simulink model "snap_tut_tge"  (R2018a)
settings: Solver=VariableStepDiscrete  StartTime=0.0  StopTime=50000  RelTol=1e-3
undefined symbols (not defined in the file): bad_frame, Bit, Both, bram, c, cnt_rst, core_rst, d, data, data_in, eof, eof_in, Falling, hex2dec, ip, ip_in, led, led_rx, led_tx, led_up, link_up, Location, Lower, Minimum_Area, notused, out, overrun, reg, Rising, ROACH2, sfp, SNAP, tx_full, tx_over, Unsigned, Upper, valid, valid_in, Width, xc7k160t
libraries: xbsIndex_r4 x1201, casper_library_misc x9, xps_library x5
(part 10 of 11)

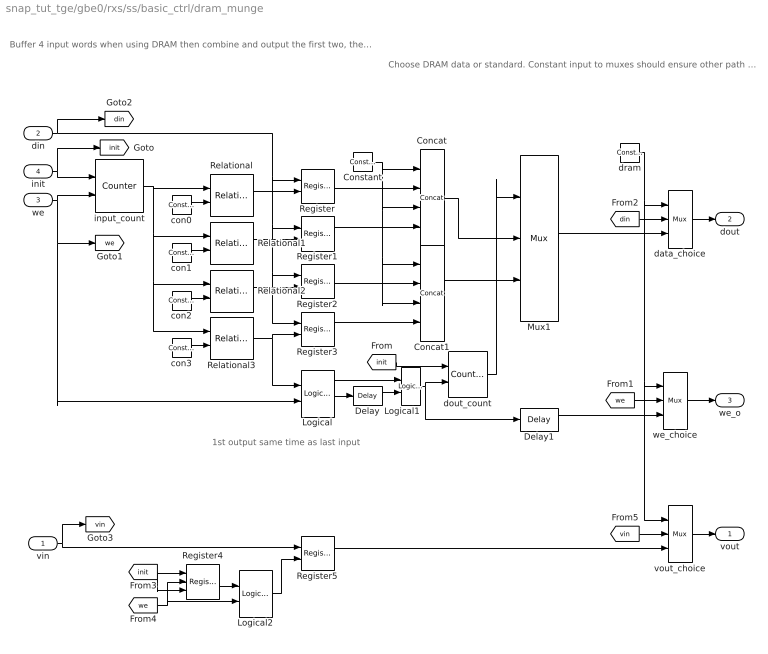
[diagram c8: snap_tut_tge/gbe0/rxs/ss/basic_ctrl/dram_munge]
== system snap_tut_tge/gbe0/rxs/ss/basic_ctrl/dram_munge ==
  note: 1st output same time as last input
  note: Choose DRAM data or standard. Constant input to muxes should ensure other path optimised away
  note: Buffer 4 input words when using DRAM then combine and output the first two, then second. Ensures that a full burst goes through every time so that status register records number of bytes fully in DRAM
  vin : Inport
  din : Inport  Port=2
  we : Inport  Port=3
  init : Inport  Port=4
  Concat : xbsIndex_r4/Concat  num_inputs=4  dbl_ovrd=off  block_type=concat
  Concat1 : xbsIndex_r4/Concat  num_inputs=4  dbl_ovrd=off  block_type=concat
  Constant : xbsIndex_r4/Constant  const=0  gui_display_data_type=Fixed-point  arith_type=Unsigned  n_bits=8  bin_pt=0  preci_type=Single  exp_width=8  frac_width=24  explicit_period=on  period=1  equ=P=C  opselect=C  inp2=PCIN>>17  opr=+  inp1=P  carry=CIN  dbl_ovrd=off  block_type=constant
  Delay : xbsIndex_r4/Delay  rst=off  infoeditControl=Selection of Reset will increase slice count due to use of real FFs and instead of SRLs  en=off  latency=1  reg_retiming=off  dbl_ovrd=off  block_type=delay
  Delay1 : xbsIndex_r4/Delay  rst=off  infoeditControl=Selection of Reset will increase slice count due to use of real FFs and instead of SRLs  en=off  latency=1  reg_retiming=off  dbl_ovrd=off  block_type=delay
  Logical : xbsIndex_r4/Logical  logical_function=AND  inputs=2  en=off  latency=1  precision=Full  arith_type=Unsigned  n_bits=16  bin_pt=0  align_bp=on  dbl_ovrd=off  block_type=logical
  Logical1 : xbsIndex_r4/Logical  logical_function=OR  inputs=2  en=off  latency=0  precision=Full  arith_type=Unsigned  n_bits=16  bin_pt=0  align_bp=on  dbl_ovrd=off  block_type=logical
  Logical2 : xbsIndex_r4/Logical  logical_function=AND  inputs=2  en=off  latency=0  precision=Full  arith_type=Unsigned  n_bits=16  bin_pt=0  align_bp=on  dbl_ovrd=off  block_type=logical
  Mux1 : xbsIndex_r4/Mux  inputs=2  en=off  latency=1  precision=Full  arith_type=Unsigned  n_bits=16  bin_pt=14  quantization=Truncate  overflow=Wrap  dbl_ovrd=off  block_type=mux
  Register{,1..3,5} (5 alike) : xbsIndex_r4/Register  init=0  rst=off  en=on  dbl_ovrd=off  block_type=register
  Register4 : xbsIndex_r4/Register  init=0  rst=on  en=on  dbl_ovrd=off  block_type=register
  Relational{,1..3} (4 alike) : xbsIndex_r4/Relational  mode=a=b  op_type=Bool  en=off  latency=0  dbl_ovrd=off  block_type=relational
  con0 : xbsIndex_r4/Constant  const=0  gui_display_data_type=Fixed-point  arith_type=Unsigned  n_bits=2  bin_pt=0  preci_type=Single  exp_width=8  frac_width=24  explicit_period=on  period=1  equ=P=C  opselect=C  inp2=PCIN>>17  opr=+  inp1=P  carry=CIN  dbl_ovrd=off  block_type=constant
  con1 : xbsIndex_r4/Constant  const=1  gui_display_data_type=Fixed-point  arith_type=Unsigned  n_bits=2  bin_pt=0  preci_type=Single  exp_width=8  frac_width=24  explicit_period=on  period=1  equ=P=C  opselect=C  inp2=PCIN>>17  opr=+  inp1=P  carry=CIN  dbl_ovrd=off  block_type=constant
  con2 : xbsIndex_r4/Constant  const=2  gui_display_data_type=Fixed-point  arith_type=Unsigned  n_bits=2  bin_pt=0  preci_type=Single  exp_width=8  frac_width=24  explicit_period=on  period=1  equ=P=C  opselect=C  inp2=PCIN>>17  opr=+  inp1=P  carry=CIN  dbl_ovrd=off  block_type=constant
  con3 : xbsIndex_r4/Constant  const=3  gui_display_data_type=Fixed-point  arith_type=Unsigned  n_bits=2  bin_pt=0  preci_type=Single  exp_width=8  frac_width=24  explicit_period=on  period=1  equ=P=C  opselect=C  inp2=PCIN>>17  opr=+  inp1=P  carry=CIN  dbl_ovrd=off  block_type=constant
  data_choice : xbsIndex_r4/Mux  inputs=2  en=off  latency=0  precision=User Defined  arith_type=Unsigned  n_bits=128  bin_pt=0  quantization=Truncate  overflow=Wrap  dbl_ovrd=off  block_type=mux
  dout_count : xbsIndex_r4/Counter  cnt_type=Free Running  cnt_to=Inf  operation=Up  start_count=0  cnt_by_val=1  arith_type=Unsigned  n_bits=1  bin_pt=0  load_pin=off  rst=on  en=on  explicit_period=on  period=1  use_behavioral_HDL=off  implementation=Fabric  dbl_ovrd=off  block_type=counter
  dram : xbsIndex_r4/Constant  const=0  gui_display_data_type=Fixed-point  arith_type=Boolean  n_bits=16  bin_pt=14  preci_type=Single  exp_width=8  frac_width=24  explicit_period=on  period=1  equ=P=C  opselect=C  inp2=PCIN>>17  opr=+  inp1=P  carry=CIN  dbl_ovrd=off  block_type=constant
  input_count : xbsIndex_r4/Counter  cnt_type=Free Running  cnt_to=Inf  operation=Up  start_count=0  cnt_by_val=1  arith_type=Unsigned  n_bits=2  bin_pt=0  load_pin=off  rst=on  en=on  explicit_period=on  period=1  use_behavioral_HDL=off  implementation=Fabric  dbl_ovrd=off  block_type=counter
  vout_choice : xbsIndex_r4/Mux  inputs=2  en=off  latency=0  precision=Full  arith_type=Unsigned  n_bits=16  bin_pt=14  quantization=Truncate  overflow=Wrap  dbl_ovrd=off  block_type=mux
  we_choice : xbsIndex_r4/Mux  inputs=2  en=off  latency=0  precision=Full  arith_type=Unsigned  n_bits=16  bin_pt=14  quantization=Truncate  overflow=Wrap  dbl_ovrd=off  block_type=mux
  vout : Outport
  dout : Outport  Port=2
  we_o : Outport  Port=3
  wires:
  Register3/1 -> Concat1/4
  Register2/1 -> Concat1/2
  Constant/1 -> Concat1/3, Concat1/1, Concat/3, Concat/1
  Register1/1 -> Concat/4
  Register/1 -> Concat/2
  [vin] -> vout_choice/2
  Register5/1 -> vout_choice/3
  vout_choice/1 -> vout/1
  Logical2/1 -> Register5/2
  [we] -> Logical2/2, Register4/2
  vin/1 -> [vin], Register5/1
  Register4/1 -> Logical2/1
  [init] -> Register4/3, Register4/1
  dram/1 -> vout_choice/1, we_choice/1, data_choice/1
  [din] -> data_choice/2
  Mux1/1 -> data_choice/3
  [we] -> we_choice/2
  Delay1/1 -> we_choice/3
  we_choice/1 -> we_o/1
  dout_count/1 -> Mux1/1
  [init] -> dout_count/1
  Logical1/1 -> Delay1/1, dout_count/2
  Concat1/1 -> Mux1/3
  Concat/1 -> Mux1/2
  Delay/1 -> Logical1/2
  Logical/1 -> Logical1/1, Delay/1
  Relational3/1 -> Logical/1, Register3/2
  Relational2/1 -> Register2/2
  Relational1/1 -> Register1/2
  Relational/1 -> Register/2
  con3/1 -> Relational3/2
  con2/1 -> Relational2/2
  con1/1 -> Relational1/2
  con0/1 -> Relational/2
  input_count/1 -> Relational3/1, Relational2/1, Relational1/1, Relational/1
  din/1 -> [din], Register3/1, Register2/1, Register1/1, Register/1
  we/1 -> [we], Logical/2, input_count/2
  init/1 -> [init], input_count/1
  data_choice/1 -> dout/1

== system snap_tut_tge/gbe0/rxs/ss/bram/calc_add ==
  note: If reading/writing words smaller than 32 bits, change address so that addressing is big endian instead of little, otherwise pass through
  note: Use behavioural HDL so that gets optimised to minimum logic
  in : Inport
  add_sub : xbsIndex_r4/AddSub  mode=Subtraction  use_carryin=off  use_carryout=off  en=off  latency=0  precision=User Defined  arith_type=Unsigned  n_bits=max(1, log2(32/data_width))  bin_pt=0  quantization=Truncate  overflow=Wrap  use_behavioral_HDL=on  hw_selection=Fabric  pipelined=off  dbl_ovrd=off  block_type=addsub
  concat : xbsIndex_r4/Concat  num_inputs=2  dbl_ovrd=off  block_type=concat
  const : xbsIndex_r4/Constant  const=max(0, 32/data_width-1)  gui_display_data_type=Fixed-point  arith_type=Unsigned  n_bits=max(1, log2(32/data_width))  bin_pt=0  preci_type=Single  exp_width=8  frac_width=24  explicit_period=on  period=sample_rate  equ=P=C  opselect=C  inp2=PCIN>>17  opr=+  inp1=P  carry=CIN  dbl_ovrd=off  block_type=constant
  convert_addr : xbsIndex_r4/Convert  gui_display_data_type=Fixed-point  arith_type=Unsigned  n_bits=addr_width  bin_pt=0  float_type=Single  exp_bits=8  fraction_bits=24  quantization=Truncate  overflow=Wrap  en=off  latency=0  pipeline=off  dbl_ovrd=off  block_type=convert
  lsw : xbsIndex_r4/Slice  nbits=max(1, log2(32/data_width))  boolean_output=off  mode=Lower Bit Location + Width  bit1=0  base1=MSB of Input  bit0=0  base0=LSB of Input  dbl_ovrd=off  block_type=slice
  manipulate : xbsIndex_r4/Constant  const=min(1, floor(32/data_width) - 1)  gui_display_data_type=Fixed-point  arith_type=Unsigned  n_bits=1  bin_pt=0  preci_type=Single  exp_width=8  frac_width=24  explicit_period=on  period=sample_rate  equ=P=C  opselect=C  inp2=PCIN>>17  opr=+  inp1=P  carry=CIN  dbl_ovrd=off  block_type=constant
  msw : xbsIndex_r4/Slice  nbits=addr_width - max(1, log2(32/data_width))  boolean_output=off  mode=Upper Bit Location + Width  bit1=0  base1=MSB of Input  bit0=0  base0=LSB of Input  dbl_ovrd=off  block_type=slice
  mux : xbsIndex_r4/Mux  inputs=2  en=off  latency=0  precision=Full  arith_type=Unsigned  n_bits=16  bin_pt=14  quantization=Truncate  overflow=Wrap  dbl_ovrd=off  block_type=mux
  out : Outport
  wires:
  in/1 -> convert_addr/1
  add_sub/1 -> concat/2
  msw/1 -> concat/1
  concat/1 -> mux/3
  manipulate/1 -> mux/1
  mux/1 -> out/1
  lsw/1 -> add_sub/2
  const/1 -> add_sub/1
  convert_addr/1 -> lsw/1, msw/1, mux/2

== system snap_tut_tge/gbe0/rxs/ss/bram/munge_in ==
  din : Inport
  join : Subsystem  AncestorBlock=casper_library_flow_control/bus_create  mask(bus_create){inputNum=4}
      mask prompts: inputNum "Number of inputs:"
      mask init:
      | bus_create_init(gcb,...
      |     'inputNum', inputNum);
  reinterpret : xbsIndex_r4/Reinterpret  force_arith_type=on  arith_type=Unsigned  force_bin_pt=on  bin_pt=0  block_type=reinterpret
  reinterpret_out : xbsIndex_r4/Reinterpret  force_arith_type=on  arith_type=Unsigned  force_bin_pt=on  bin_pt=0  block_type=reinterpret
  split : Subsystem  AncestorBlock=casper_library_flow_control/bus_expand  mask(bus_expand){mode=divisions of arbitrary size, outputNum=1, outputWidth=[32 32 32 32], outputBinaryPt=[0 0 0 0], outputArithmeticType=[0 0 0 0], show_format=off, outputToWorkspace=off, variablePrefix=out, outputToModelAsWell=on}
      mask prompts: outputNum "Number of outputs:"; outputWidth "Output width [msb ... lsb]:"; outputBinaryPt "Output binary point position [msb ... lsb]:"; outputArithmeticType "Output arithmetic type (ufix=0, fix=1, bool=2) [msb ... lsb]:"; show_format "Print format string?"; outputToWorkspace "Output to workspace?"; variablePrefix "Variable name prefix:"; outputToModelAsWell "Output to model as well?"
      mask help: Expands a 'bus' made using a bus_create or Xilinx concat block. The input will be divided into the specified number of outputs with the specified arithmetic types. Divisions are made from most significant bit.
      mask init:
      | bus_expand_init(gcb,...
      |     'mode', mode, ...
      |     'outputNum', outputNum, ...
      |     'outputWidth', outputWidth, ...
      |     'outputBinaryPt', outputBinaryPt, ...
      |     'outputArithmeticType', outputArithmeticType, ...
      |     'show_format', show_format, ...
      |     'outputToWorkspace', outputToWorkspace, ...
      |     'variablePrefix', variablePrefix, ...
      |     'outputToModelAsWell', outputToModelAsWell);
  dout : Outport
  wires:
  reinterpret_out/1 -> dout/1
  din/1 -> reinterpret/1
  reinterpret/1 -> split/1(bus_in)
  join/1(bus_out) -> reinterpret_out/1
  split/4(lsb_out1) -> join/1(in1)
  split/3(out2) -> join/2(in2)
  split/2(out3) -> join/3(in3)
  split/1(msb_out4) -> join/4(in4)

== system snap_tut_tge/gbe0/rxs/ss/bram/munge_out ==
  din : Inport
  join : Subsystem  AncestorBlock=casper_library_flow_control/bus_create  mask(bus_create){inputNum=4}
      mask prompts: inputNum "Number of inputs:"
      mask init:
      | bus_create_init(gcb,...
      |     'inputNum', inputNum);
  reinterpret : xbsIndex_r4/Reinterpret  force_arith_type=on  arith_type=Unsigned  force_bin_pt=on  bin_pt=0  block_type=reinterpret
  reinterpret_out : xbsIndex_r4/Reinterpret  force_arith_type=on  arith_type=Unsigned  force_bin_pt=on  bin_pt=0  block_type=reinterpret
  split : Subsystem  AncestorBlock=casper_library_flow_control/bus_expand  mask(bus_expand){mode=divisions of arbitrary size, outputNum=1, outputWidth=[32 32 32 32], outputBinaryPt=[0 0 0 0], outputArithmeticType=[0 0 0 0], show_format=off, outputToWorkspace=off, variablePrefix=out, outputToModelAsWell=on}
      mask prompts: outputNum "Number of outputs:"; outputWidth "Output width [msb ... lsb]:"; outputBinaryPt "Output binary point position [msb ... lsb]:"; outputArithmeticType "Output arithmetic type (ufix=0, fix=1, bool=2) [msb ... lsb]:"; show_format "Print format string?"; outputToWorkspace "Output to workspace?"; variablePrefix "Variable name prefix:"; outputToModelAsWell "Output to model as well?"
      mask help: Expands a 'bus' made using a bus_create or Xilinx concat block. The input will be divided into the specified number of outputs with the specified arithmetic types. Divisions are made from most significant bit.
      mask init:
      | bus_expand_init(gcb,...
      |     'mode', mode, ...
      |     'outputNum', outputNum, ...
      |     'outputWidth', outputWidth, ...
      |     'outputBinaryPt', outputBinaryPt, ...
      |     'outputArithmeticType', outputArithmeticType, ...
      |     'show_format', show_format, ...
      |     'outputToWorkspace', outputToWorkspace, ...
      |     'variablePrefix', variablePrefix, ...
      |     'outputToModelAsWell', outputToModelAsWell);
  dout : Outport
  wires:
  reinterpret_out/1 -> dout/1
  din/1 -> reinterpret/1
  reinterpret/1 -> split/1(bus_in)
  join/1(bus_out) -> reinterpret_out/1
  split/4(lsb_out1) -> join/1(in1)
  split/3(out2) -> join/2(in2)
  split/2(out3) -> join/3(in3)
  split/1(msb_out4) -> join/4(in4)

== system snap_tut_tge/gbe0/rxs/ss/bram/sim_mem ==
  addr : Inport
  data : Inport  Port=2
  we : Inport  Port=3
  Data Type Conversion : DataTypeConversion  OutDataTypeStr=single
  Data Type Conversion1 : DataTypeConversion  OutDataTypeStr=double
  Data Type Conversion2 : DataTypeConversion  OutDataTypeStr=boolean
  sfunc : M-S-Function  FunctionName=shared_bram_sim_sfunc  Parameters=depth_bits, latency, init_vals  mask{depth_bits=addr_width, latency=csp_latency, init_vals=init_vals}
      mask prompts: depth_bits "Depth (2^?):"; latency "Latency (>=1):"; init_vals "Initial values:"
  sim_addr : xbsIndex_r4/Gateway Out  inherit_from_input=off  hdl_port=off  rows=1  columns=1  UseAsDAC=off  DACChannel='1'  interface=None  automatic_assignment=on  address_offset=hex2dec('00')  intf_name=''  intf_description=''  timing_constraint=None  locs_specified=off  LOCs={}  io_standard={}  block_type=gatewayout
  sim_data : xbsIndex_r4/Gateway Out  inherit_from_input=off  hdl_port=off  rows=1  columns=1  UseAsDAC=off  DACChannel='1'  interface=None  automatic_assignment=on  address_offset=hex2dec('00')  intf_name=''  intf_description=''  timing_constraint=None  locs_specified=off  LOCs={}  io_standard={}  block_type=gatewayout
  sim_we : xbsIndex_r4/Gateway Out  inherit_from_input=off  hdl_port=off  rows=1  columns=1  UseAsDAC=off  DACChannel='1'  interface=None  automatic_assignment=on  address_offset=hex2dec('00')  intf_name=''  intf_description=''  timing_constraint=None  locs_specified=off  LOCs={}  io_standard={}  block_type=gatewayout
  data_out : Outport
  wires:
  addr/1 -> sim_addr/1
  data/1 -> sim_data/1
  we/1 -> sim_we/1
  sim_addr/1 -> Data Type Conversion/1
  sim_data/1 -> Data Type Conversion1/1
  sim_we/1 -> Data Type Conversion2/1
  Data Type Conversion/1 -> sfunc/1  "addr"
  Data Type Conversion1/1 -> sfunc/2  "data_in"
  Data Type Conversion2/1 -> sfunc/3  "we"
  sfunc/1 -> data_out/1  "output"

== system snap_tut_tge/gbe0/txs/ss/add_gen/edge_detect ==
  in : Inport
  Delay : xbsIndex_r4/Delay  rst=off  infoeditControl=Selection of Reset will increase slice count due to use of real FFs and instead of SRLs  en=off  latency=1  reg_retiming=off  dbl_ovrd=off  block_type=delay
  Inverter : xbsIndex_r4/Inverter  en=off  latency=0  dbl_ovrd=off  block_type=inv
  edge_op : xbsIndex_r4/Logical  logical_function=XNOR  inputs=2  en=off  latency=0  precision=Full  arith_type=Unsigned  n_bits=8  bin_pt=2  align_bp=on  dbl_ovrd=off  block_type=logical
  out : Outport
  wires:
  Delay/1 -> edge_op/2
  in/1 -> Delay/1, Inverter/1
  edge_op/1 -> out/1
  Inverter/1 -> edge_op/1

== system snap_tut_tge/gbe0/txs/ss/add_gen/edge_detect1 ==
  in : Inport
  Delay : xbsIndex_r4/Delay  rst=off  infoeditControl=Selection of Reset will increase slice count due to use of real FFs and instead of SRLs  en=off  latency=1  reg_retiming=off  dbl_ovrd=off  block_type=delay
  Inverter : xbsIndex_r4/Inverter  en=off  latency=0  dbl_ovrd=off  block_type=inv
  edge_op : xbsIndex_r4/Logical  logical_function=XNOR  inputs=2  en=off  latency=0  precision=Full  arith_type=Unsigned  n_bits=8  bin_pt=2  align_bp=on  dbl_ovrd=off  block_type=logical
  out : Outport
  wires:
  Inverter/1 -> edge_op/1
  edge_op/1 -> out/1
  in/1 -> Inverter/1, Delay/1
  Delay/1 -> edge_op/2

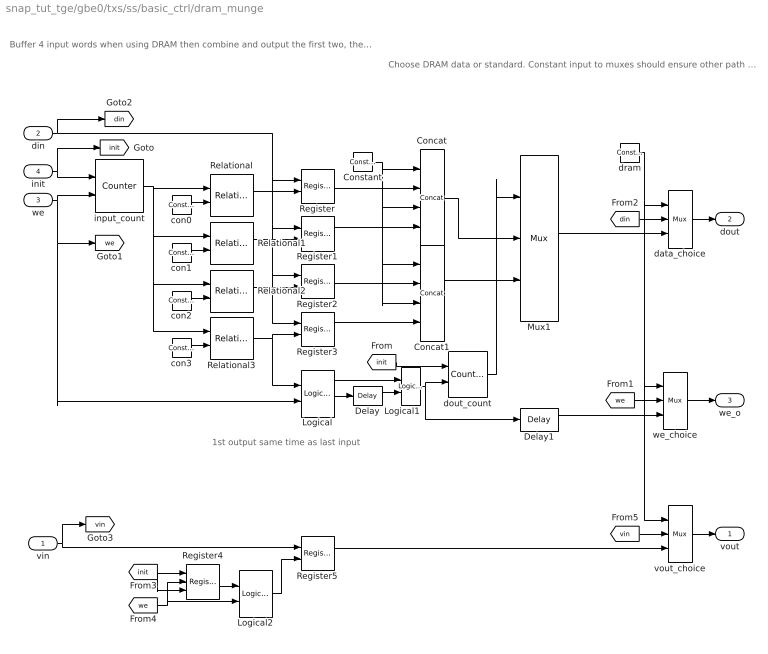
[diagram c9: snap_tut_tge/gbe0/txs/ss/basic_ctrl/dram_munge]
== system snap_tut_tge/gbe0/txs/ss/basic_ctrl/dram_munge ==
  note: 1st output same time as last input
  note: Choose DRAM data or standard. Constant input to muxes should ensure other path optimised away
  note: Buffer 4 input words when using DRAM then combine and output the first two, then second. Ensures that a full burst goes through every time so that status register records number of bytes fully in DRAM
  vin : Inport
  din : Inport  Port=2
  we : Inport  Port=3
  init : Inport  Port=4
  Concat : xbsIndex_r4/Concat  num_inputs=4  dbl_ovrd=off  block_type=concat
  Concat1 : xbsIndex_r4/Concat  num_inputs=4  dbl_ovrd=off  block_type=concat
  Constant : xbsIndex_r4/Constant  const=0  gui_display_data_type=Fixed-point  arith_type=Unsigned  n_bits=8  bin_pt=0  preci_type=Single  exp_width=8  frac_width=24  explicit_period=on  period=1  equ=P=C  opselect=C  inp2=PCIN>>17  opr=+  inp1=P  carry=CIN  dbl_ovrd=off  block_type=constant
  Delay : xbsIndex_r4/Delay  rst=off  infoeditControl=Selection of Reset will increase slice count due to use of real FFs and instead of SRLs  en=off  latency=1  reg_retiming=off  dbl_ovrd=off  block_type=delay
  Delay1 : xbsIndex_r4/Delay  rst=off  infoeditControl=Selection of Reset will increase slice count due to use of real FFs and instead of SRLs  en=off  latency=1  reg_retiming=off  dbl_ovrd=off  block_type=delay
  Logical : xbsIndex_r4/Logical  logical_function=AND  inputs=2  en=off  latency=1  precision=Full  arith_type=Unsigned  n_bits=16  bin_pt=0  align_bp=on  dbl_ovrd=off  block_type=logical
  Logical1 : xbsIndex_r4/Logical  logical_function=OR  inputs=2  en=off  latency=0  precision=Full  arith_type=Unsigned  n_bits=16  bin_pt=0  align_bp=on  dbl_ovrd=off  block_type=logical
  Logical2 : xbsIndex_r4/Logical  logical_function=AND  inputs=2  en=off  latency=0  precision=Full  arith_type=Unsigned  n_bits=16  bin_pt=0  align_bp=on  dbl_ovrd=off  block_type=logical
  Mux1 : xbsIndex_r4/Mux  inputs=2  en=off  latency=1  precision=Full  arith_type=Unsigned  n_bits=16  bin_pt=14  quantization=Truncate  overflow=Wrap  dbl_ovrd=off  block_type=mux
  Register{,1..3,5} (5 alike) : xbsIndex_r4/Register  init=0  rst=off  en=on  dbl_ovrd=off  block_type=register
  Register4 : xbsIndex_r4/Register  init=0  rst=on  en=on  dbl_ovrd=off  block_type=register
  Relational{,1..3} (4 alike) : xbsIndex_r4/Relational  mode=a=b  op_type=Bool  en=off  latency=0  dbl_ovrd=off  block_type=relational
  con0 : xbsIndex_r4/Constant  const=0  gui_display_data_type=Fixed-point  arith_type=Unsigned  n_bits=2  bin_pt=0  preci_type=Single  exp_width=8  frac_width=24  explicit_period=on  period=1  equ=P=C  opselect=C  inp2=PCIN>>17  opr=+  inp1=P  carry=CIN  dbl_ovrd=off  block_type=constant
  con1 : xbsIndex_r4/Constant  const=1  gui_display_data_type=Fixed-point  arith_type=Unsigned  n_bits=2  bin_pt=0  preci_type=Single  exp_width=8  frac_width=24  explicit_period=on  period=1  equ=P=C  opselect=C  inp2=PCIN>>17  opr=+  inp1=P  carry=CIN  dbl_ovrd=off  block_type=constant
  con2 : xbsIndex_r4/Constant  const=2  gui_display_data_type=Fixed-point  arith_type=Unsigned  n_bits=2  bin_pt=0  preci_type=Single  exp_width=8  frac_width=24  explicit_period=on  period=1  equ=P=C  opselect=C  inp2=PCIN>>17  opr=+  inp1=P  carry=CIN  dbl_ovrd=off  block_type=constant
  con3 : xbsIndex_r4/Constant  const=3  gui_display_data_type=Fixed-point  arith_type=Unsigned  n_bits=2  bin_pt=0  preci_type=Single  exp_width=8  frac_width=24  explicit_period=on  period=1  equ=P=C  opselect=C  inp2=PCIN>>17  opr=+  inp1=P  carry=CIN  dbl_ovrd=off  block_type=constant
  data_choice : xbsIndex_r4/Mux  inputs=2  en=off  latency=0  precision=User Defined  arith_type=Unsigned  n_bits=128  bin_pt=0  quantization=Truncate  overflow=Wrap  dbl_ovrd=off  block_type=mux
  dout_count : xbsIndex_r4/Counter  cnt_type=Free Running  cnt_to=Inf  operation=Up  start_count=0  cnt_by_val=1  arith_type=Unsigned  n_bits=1  bin_pt=0  load_pin=off  rst=on  en=on  explicit_period=on  period=1  use_behavioral_HDL=off  implementation=Fabric  dbl_ovrd=off  block_type=counter
  dram : xbsIndex_r4/Constant  const=0  gui_display_data_type=Fixed-point  arith_type=Boolean  n_bits=16  bin_pt=14  preci_type=Single  exp_width=8  frac_width=24  explicit_period=on  period=1  equ=P=C  opselect=C  inp2=PCIN>>17  opr=+  inp1=P  carry=CIN  dbl_ovrd=off  block_type=constant
  input_count : xbsIndex_r4/Counter  cnt_type=Free Running  cnt_to=Inf  operation=Up  start_count=0  cnt_by_val=1  arith_type=Unsigned  n_bits=2  bin_pt=0  load_pin=off  rst=on  en=on  explicit_period=on  period=1  use_behavioral_HDL=off  implementation=Fabric  dbl_ovrd=off  block_type=counter
  vout_choice : xbsIndex_r4/Mux  inputs=2  en=off  latency=0  precision=Full  arith_type=Unsigned  n_bits=16  bin_pt=14  quantization=Truncate  overflow=Wrap  dbl_ovrd=off  block_type=mux
  we_choice : xbsIndex_r4/Mux  inputs=2  en=off  latency=0  precision=Full  arith_type=Unsigned  n_bits=16  bin_pt=14  quantization=Truncate  overflow=Wrap  dbl_ovrd=off  block_type=mux
  vout : Outport
  dout : Outport  Port=2
  we_o : Outport  Port=3
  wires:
  Register3/1 -> Concat1/4
  Register2/1 -> Concat1/2
  Constant/1 -> Concat1/3, Concat1/1, Concat/3, Concat/1
  Register1/1 -> Concat/4
  Register/1 -> Concat/2
  [vin] -> vout_choice/2
  Register5/1 -> vout_choice/3
  vout_choice/1 -> vout/1
  Logical2/1 -> Register5/2
  [we] -> Logical2/2, Register4/2
  vin/1 -> [vin], Register5/1
  Register4/1 -> Logical2/1
  [init] -> Register4/3, Register4/1
  dram/1 -> vout_choice/1, we_choice/1, data_choice/1
  [din] -> data_choice/2
  Mux1/1 -> data_choice/3
  [we] -> we_choice/2
  Delay1/1 -> we_choice/3
  we_choice/1 -> we_o/1
  dout_count/1 -> Mux1/1
  [init] -> dout_count/1
  Logical1/1 -> Delay1/1, dout_count/2
  Concat1/1 -> Mux1/3
  Concat/1 -> Mux1/2
  Delay/1 -> Logical1/2
  Logical/1 -> Logical1/1, Delay/1
  Relational3/1 -> Logical/1, Register3/2
  Relational2/1 -> Register2/2
  Relational1/1 -> Register1/2
  Relational/1 -> Register/2
  con3/1 -> Relational3/2
  con2/1 -> Relational2/2
  con1/1 -> Relational1/2
  con0/1 -> Relational/2
  input_count/1 -> Relational3/1, Relational2/1, Relational1/1, Relational/1
  din/1 -> [din], Register3/1, Register2/1, Register1/1, Register/1
  we/1 -> [we], Logical/2, input_count/2
  init/1 -> [init], input_count/1
  data_choice/1 -> dout/1

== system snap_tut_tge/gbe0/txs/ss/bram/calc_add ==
  note: If reading/writing words smaller than 32 bits, change address so that addressing is big endian instead of little, otherwise pass through
  note: Use behavioural HDL so that gets optimised to minimum logic
  in : Inport
  add_sub : xbsIndex_r4/AddSub  mode=Subtraction  use_carryin=off  use_carryout=off  en=off  latency=0  precision=User Defined  arith_type=Unsigned  n_bits=max(1, log2(32/data_width))  bin_pt=0  quantization=Truncate  overflow=Wrap  use_behavioral_HDL=on  hw_selection=Fabric  pipelined=off  dbl_ovrd=off  block_type=addsub
  concat : xbsIndex_r4/Concat  num_inputs=2  dbl_ovrd=off  block_type=concat
  const : xbsIndex_r4/Constant  const=max(0, 32/data_width-1)  gui_display_data_type=Fixed-point  arith_type=Unsigned  n_bits=max(1, log2(32/data_width))  bin_pt=0  preci_type=Single  exp_width=8  frac_width=24  explicit_period=on  period=sample_rate  equ=P=C  opselect=C  inp2=PCIN>>17  opr=+  inp1=P  carry=CIN  dbl_ovrd=off  block_type=constant
  convert_addr : xbsIndex_r4/Convert  gui_display_data_type=Fixed-point  arith_type=Unsigned  n_bits=addr_width  bin_pt=0  float_type=Single  exp_bits=8  fraction_bits=24  quantization=Truncate  overflow=Wrap  en=off  latency=0  pipeline=off  dbl_ovrd=off  block_type=convert
  lsw : xbsIndex_r4/Slice  nbits=max(1, log2(32/data_width))  boolean_output=off  mode=Lower Bit Location + Width  bit1=0  base1=MSB of Input  bit0=0  base0=LSB of Input  dbl_ovrd=off  block_type=slice
  manipulate : xbsIndex_r4/Constant  const=min(1, floor(32/data_width) - 1)  gui_display_data_type=Fixed-point  arith_type=Unsigned  n_bits=1  bin_pt=0  preci_type=Single  exp_width=8  frac_width=24  explicit_period=on  period=sample_rate  equ=P=C  opselect=C  inp2=PCIN>>17  opr=+  inp1=P  carry=CIN  dbl_ovrd=off  block_type=constant
  msw : xbsIndex_r4/Slice  nbits=addr_width - max(1, log2(32/data_width))  boolean_output=off  mode=Upper Bit Location + Width  bit1=0  base1=MSB of Input  bit0=0  base0=LSB of Input  dbl_ovrd=off  block_type=slice
  mux : xbsIndex_r4/Mux  inputs=2  en=off  latency=0  precision=Full  arith_type=Unsigned  n_bits=16  bin_pt=14  quantization=Truncate  overflow=Wrap  dbl_ovrd=off  block_type=mux
  out : Outport
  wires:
  in/1 -> convert_addr/1
  add_sub/1 -> concat/2
  msw/1 -> concat/1
  concat/1 -> mux/3
  manipulate/1 -> mux/1
  mux/1 -> out/1
  lsw/1 -> add_sub/2
  const/1 -> add_sub/1
  convert_addr/1 -> lsw/1, msw/1, mux/2

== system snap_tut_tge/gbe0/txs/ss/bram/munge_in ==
  din : Inport
  join : Subsystem  AncestorBlock=casper_library_flow_control/bus_create  mask(bus_create){inputNum=4}
      mask prompts: inputNum "Number of inputs:"
      mask init:
      | bus_create_init(gcb,...
      |     'inputNum', inputNum);
  reinterpret : xbsIndex_r4/Reinterpret  force_arith_type=on  arith_type=Unsigned  force_bin_pt=on  bin_pt=0  block_type=reinterpret
  reinterpret_out : xbsIndex_r4/Reinterpret  force_arith_type=on  arith_type=Unsigned  force_bin_pt=on  bin_pt=0  block_type=reinterpret
  split : Subsystem  AncestorBlock=casper_library_flow_control/bus_expand  mask(bus_expand){mode=divisions of arbitrary size, outputNum=1, outputWidth=[32 32 32 32], outputBinaryPt=[0 0 0 0], outputArithmeticType=[0 0 0 0], show_format=off, outputToWorkspace=off, variablePrefix=out, outputToModelAsWell=on}
      mask prompts: outputNum "Number of outputs:"; outputWidth "Output width [msb ... lsb]:"; outputBinaryPt "Output binary point position [msb ... lsb]:"; outputArithmeticType "Output arithmetic type (ufix=0, fix=1, bool=2) [msb ... lsb]:"; show_format "Print format string?"; outputToWorkspace "Output to workspace?"; variablePrefix "Variable name prefix:"; outputToModelAsWell "Output to model as well?"
      mask help: Expands a 'bus' made using a bus_create or Xilinx concat block. The input will be divided into the specified number of outputs with the specified arithmetic types. Divisions are made from most significant bit.
      mask init:
      | bus_expand_init(gcb,...
      |     'mode', mode, ...
      |     'outputNum', outputNum, ...
      |     'outputWidth', outputWidth, ...
      |     'outputBinaryPt', outputBinaryPt, ...
      |     'outputArithmeticType', outputArithmeticType, ...
      |     'show_format', show_format, ...
      |     'outputToWorkspace', outputToWorkspace, ...
      |     'variablePrefix', variablePrefix, ...
      |     'outputToModelAsWell', outputToModelAsWell);
  dout : Outport
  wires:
  reinterpret_out/1 -> dout/1
  din/1 -> reinterpret/1
  reinterpret/1 -> split/1(bus_in)
  join/1(bus_out) -> reinterpret_out/1
  split/4(lsb_out1) -> join/1(in1)
  split/3(out2) -> join/2(in2)
  split/2(out3) -> join/3(in3)
  split/1(msb_out4) -> join/4(in4)

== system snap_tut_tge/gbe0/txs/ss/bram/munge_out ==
  din : Inport
  join : Subsystem  AncestorBlock=casper_library_flow_control/bus_create  mask(bus_create){inputNum=4}
      mask prompts: inputNum "Number of inputs:"
      mask init:
      | bus_create_init(gcb,...
      |     'inputNum', inputNum);
  reinterpret : xbsIndex_r4/Reinterpret  force_arith_type=on  arith_type=Unsigned  force_bin_pt=on  bin_pt=0  block_type=reinterpret
  reinterpret_out : xbsIndex_r4/Reinterpret  force_arith_type=on  arith_type=Unsigned  force_bin_pt=on  bin_pt=0  block_type=reinterpret
  split : Subsystem  AncestorBlock=casper_library_flow_control/bus_expand  mask(bus_expand){mode=divisions of arbitrary size, outputNum=1, outputWidth=[32 32 32 32], outputBinaryPt=[0 0 0 0], outputArithmeticType=[0 0 0 0], show_format=off, outputToWorkspace=off, variablePrefix=out, outputToModelAsWell=on}
      mask prompts: outputNum "Number of outputs:"; outputWidth "Output width [msb ... lsb]:"; outputBinaryPt "Output binary point position [msb ... lsb]:"; outputArithmeticType "Output arithmetic type (ufix=0, fix=1, bool=2) [msb ... lsb]:"; show_format "Print format string?"; outputToWorkspace "Output to workspace?"; variablePrefix "Variable name prefix:"; outputToModelAsWell "Output to model as well?"
      mask help: Expands a 'bus' made using a bus_create or Xilinx concat block. The input will be divided into the specified number of outputs with the specified arithmetic types. Divisions are made from most significant bit.
      mask init:
      | bus_expand_init(gcb,...
      |     'mode', mode, ...
      |     'outputNum', outputNum, ...
      |     'outputWidth', outputWidth, ...
      |     'outputBinaryPt', outputBinaryPt, ...
      |     'outputArithmeticType', outputArithmeticType, ...
      |     'show_format', show_format, ...
      |     'outputToWorkspace', outputToWorkspace, ...
      |     'variablePrefix', variablePrefix, ...
      |     'outputToModelAsWell', outputToModelAsWell);
  dout : Outport
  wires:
  reinterpret_out/1 -> dout/1
  din/1 -> reinterpret/1
  reinterpret/1 -> split/1(bus_in)
  join/1(bus_out) -> reinterpret_out/1
  split/4(lsb_out1) -> join/1(in1)
  split/3(out2) -> join/2(in2)
  split/2(out3) -> join/3(in3)
  split/1(msb_out4) -> join/4(in4)

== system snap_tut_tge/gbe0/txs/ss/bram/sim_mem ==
  addr : Inport
  data : Inport  Port=2
  we : Inport  Port=3
  Data Type Conversion : DataTypeConversion  OutDataTypeStr=single
  Data Type Conversion1 : DataTypeConversion  OutDataTypeStr=double
  Data Type Conversion2 : DataTypeConversion  OutDataTypeStr=boolean
  sfunc : M-S-Function  FunctionName=shared_bram_sim_sfunc  Parameters=depth_bits, latency, init_vals  mask{depth_bits=addr_width, latency=csp_latency, init_vals=init_vals}
      mask prompts: depth_bits "Depth (2^?):"; latency "Latency (>=1):"; init_vals "Initial values:"
  sim_addr : xbsIndex_r4/Gateway Out  inherit_from_input=off  hdl_port=off  rows=1  columns=1  UseAsDAC=off  DACChannel='1'  interface=None  automatic_assignment=on  address_offset=hex2dec('00')  intf_name=''  intf_description=''  timing_constraint=None  locs_specified=off  LOCs={}  io_standard={}  block_type=gatewayout
  sim_data : xbsIndex_r4/Gateway Out  inherit_from_input=off  hdl_port=off  rows=1  columns=1  UseAsDAC=off  DACChannel='1'  interface=None  automatic_assignment=on  address_offset=hex2dec('00')  intf_name=''  intf_description=''  timing_constraint=None  locs_specified=off  LOCs={}  io_standard={}  block_type=gatewayout
  sim_we : xbsIndex_r4/Gateway Out  inherit_from_input=off  hdl_port=off  rows=1  columns=1  UseAsDAC=off  DACChannel='1'  interface=None  automatic_assignment=on  address_offset=hex2dec('00')  intf_name=''  intf_description=''  timing_constraint=None  locs_specified=off  LOCs={}  io_standard={}  block_type=gatewayout
  data_out : Outport
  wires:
  addr/1 -> sim_addr/1
  data/1 -> sim_data/1
  we/1 -> sim_we/1
  sim_addr/1 -> Data Type Conversion/1
  sim_data/1 -> Data Type Conversion1/1
  sim_we/1 -> Data Type Conversion2/1
  Data Type Conversion/1 -> sfunc/1  "addr"
  Data Type Conversion1/1 -> sfunc/2  "data_in"
  Data Type Conversion2/1 -> sfunc/3  "we"
  sfunc/1 -> data_out/1  "output"

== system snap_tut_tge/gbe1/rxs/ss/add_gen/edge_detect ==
  in : Inport
  Delay : xbsIndex_r4/Delay  rst=off  infoeditControl=Selection of Reset will increase slice count due to use of real FFs and instead of SRLs  en=off  latency=1  reg_retiming=off  dbl_ovrd=off  block_type=delay
  Inverter : xbsIndex_r4/Inverter  en=off  latency=0  dbl_ovrd=off  block_type=inv
  edge_op : xbsIndex_r4/Logical  logical_function=XNOR  inputs=2  en=off  latency=0  precision=Full  arith_type=Unsigned  n_bits=8  bin_pt=2  align_bp=on  dbl_ovrd=off  block_type=logical
  out : Outport
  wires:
  Delay/1 -> edge_op/2
  in/1 -> Delay/1, Inverter/1
  edge_op/1 -> out/1
  Inverter/1 -> edge_op/1

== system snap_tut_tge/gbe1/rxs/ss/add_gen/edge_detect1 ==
  in : Inport
  Delay : xbsIndex_r4/Delay  rst=off  infoeditControl=Selection of Reset will increase slice count due to use of real FFs and instead of SRLs  en=off  latency=1  reg_retiming=off  dbl_ovrd=off  block_type=delay
  Inverter : xbsIndex_r4/Inverter  en=off  latency=0  dbl_ovrd=off  block_type=inv
  edge_op : xbsIndex_r4/Logical  logical_function=XNOR  inputs=2  en=off  latency=0  precision=Full  arith_type=Unsigned  n_bits=8  bin_pt=2  align_bp=on  dbl_ovrd=off  block_type=logical
  out : Outport
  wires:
  Inverter/1 -> edge_op/1
  edge_op/1 -> out/1
  in/1 -> Inverter/1, Delay/1
  Delay/1 -> edge_op/2

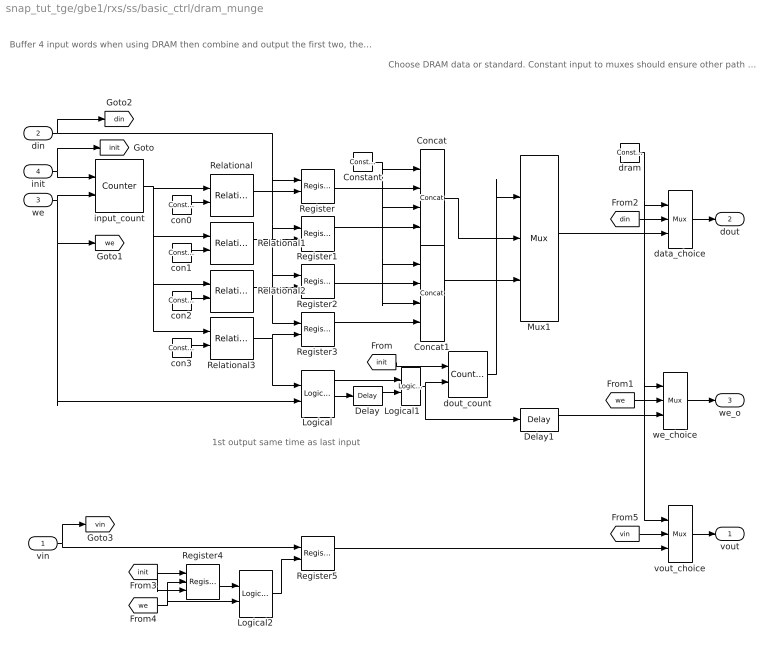
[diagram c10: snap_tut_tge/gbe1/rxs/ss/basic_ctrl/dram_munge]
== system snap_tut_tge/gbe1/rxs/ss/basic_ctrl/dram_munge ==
  note: 1st output same time as last input
  note: Choose DRAM data or standard. Constant input to muxes should ensure other path optimised away
  note: Buffer 4 input words when using DRAM then combine and output the first two, then second. Ensures that a full burst goes through every time so that status register records number of bytes fully in DRAM
  vin : Inport
  din : Inport  Port=2
  we : Inport  Port=3
  init : Inport  Port=4
  Concat : xbsIndex_r4/Concat  num_inputs=4  dbl_ovrd=off  block_type=concat
  Concat1 : xbsIndex_r4/Concat  num_inputs=4  dbl_ovrd=off  block_type=concat
  Constant : xbsIndex_r4/Constant  const=0  gui_display_data_type=Fixed-point  arith_type=Unsigned  n_bits=8  bin_pt=0  preci_type=Single  exp_width=8  frac_width=24  explicit_period=on  period=1  equ=P=C  opselect=C  inp2=PCIN>>17  opr=+  inp1=P  carry=CIN  dbl_ovrd=off  block_type=constant
  Delay : xbsIndex_r4/Delay  rst=off  infoeditControl=Selection of Reset will increase slice count due to use of real FFs and instead of SRLs  en=off  latency=1  reg_retiming=off  dbl_ovrd=off  block_type=delay
  Delay1 : xbsIndex_r4/Delay  rst=off  infoeditControl=Selection of Reset will increase slice count due to use of real FFs and instead of SRLs  en=off  latency=1  reg_retiming=off  dbl_ovrd=off  block_type=delay
  Logical : xbsIndex_r4/Logical  logical_function=AND  inputs=2  en=off  latency=1  precision=Full  arith_type=Unsigned  n_bits=16  bin_pt=0  align_bp=on  dbl_ovrd=off  block_type=logical
  Logical1 : xbsIndex_r4/Logical  logical_function=OR  inputs=2  en=off  latency=0  precision=Full  arith_type=Unsigned  n_bits=16  bin_pt=0  align_bp=on  dbl_ovrd=off  block_type=logical
  Logical2 : xbsIndex_r4/Logical  logical_function=AND  inputs=2  en=off  latency=0  precision=Full  arith_type=Unsigned  n_bits=16  bin_pt=0  align_bp=on  dbl_ovrd=off  block_type=logical
  Mux1 : xbsIndex_r4/Mux  inputs=2  en=off  latency=1  precision=Full  arith_type=Unsigned  n_bits=16  bin_pt=14  quantization=Truncate  overflow=Wrap  dbl_ovrd=off  block_type=mux
  Register{,1..3,5} (5 alike) : xbsIndex_r4/Register  init=0  rst=off  en=on  dbl_ovrd=off  block_type=register
  Register4 : xbsIndex_r4/Register  init=0  rst=on  en=on  dbl_ovrd=off  block_type=register
  Relational{,1..3} (4 alike) : xbsIndex_r4/Relational  mode=a=b  op_type=Bool  en=off  latency=0  dbl_ovrd=off  block_type=relational
  con0 : xbsIndex_r4/Constant  const=0  gui_display_data_type=Fixed-point  arith_type=Unsigned  n_bits=2  bin_pt=0  preci_type=Single  exp_width=8  frac_width=24  explicit_period=on  period=1  equ=P=C  opselect=C  inp2=PCIN>>17  opr=+  inp1=P  carry=CIN  dbl_ovrd=off  block_type=constant
  con1 : xbsIndex_r4/Constant  const=1  gui_display_data_type=Fixed-point  arith_type=Unsigned  n_bits=2  bin_pt=0  preci_type=Single  exp_width=8  frac_width=24  explicit_period=on  period=1  equ=P=C  opselect=C  inp2=PCIN>>17  opr=+  inp1=P  carry=CIN  dbl_ovrd=off  block_type=constant
  con2 : xbsIndex_r4/Constant  const=2  gui_display_data_type=Fixed-point  arith_type=Unsigned  n_bits=2  bin_pt=0  preci_type=Single  exp_width=8  frac_width=24  explicit_period=on  period=1  equ=P=C  opselect=C  inp2=PCIN>>17  opr=+  inp1=P  carry=CIN  dbl_ovrd=off  block_type=constant
  con3 : xbsIndex_r4/Constant  const=3  gui_display_data_type=Fixed-point  arith_type=Unsigned  n_bits=2  bin_pt=0  preci_type=Single  exp_width=8  frac_width=24  explicit_period=on  period=1  equ=P=C  opselect=C  inp2=PCIN>>17  opr=+  inp1=P  carry=CIN  dbl_ovrd=off  block_type=constant
  data_choice : xbsIndex_r4/Mux  inputs=2  en=off  latency=0  precision=User Defined  arith_type=Unsigned  n_bits=128  bin_pt=0  quantization=Truncate  overflow=Wrap  dbl_ovrd=off  block_type=mux
  dout_count : xbsIndex_r4/Counter  cnt_type=Free Running  cnt_to=Inf  operation=Up  start_count=0  cnt_by_val=1  arith_type=Unsigned  n_bits=1  bin_pt=0  load_pin=off  rst=on  en=on  explicit_period=on  period=1  use_behavioral_HDL=off  implementation=Fabric  dbl_ovrd=off  block_type=counter
  dram : xbsIndex_r4/Constant  const=0  gui_display_data_type=Fixed-point  arith_type=Boolean  n_bits=16  bin_pt=14  preci_type=Single  exp_width=8  frac_width=24  explicit_period=on  period=1  equ=P=C  opselect=C  inp2=PCIN>>17  opr=+  inp1=P  carry=CIN  dbl_ovrd=off  block_type=constant
  input_count : xbsIndex_r4/Counter  cnt_type=Free Running  cnt_to=Inf  operation=Up  start_count=0  cnt_by_val=1  arith_type=Unsigned  n_bits=2  bin_pt=0  load_pin=off  rst=on  en=on  explicit_period=on  period=1  use_behavioral_HDL=off  implementation=Fabric  dbl_ovrd=off  block_type=counter
  vout_choice : xbsIndex_r4/Mux  inputs=2  en=off  latency=0  precision=Full  arith_type=Unsigned  n_bits=16  bin_pt=14  quantization=Truncate  overflow=Wrap  dbl_ovrd=off  block_type=mux
  we_choice : xbsIndex_r4/Mux  inputs=2  en=off  latency=0  precision=Full  arith_type=Unsigned  n_bits=16  bin_pt=14  quantization=Truncate  overflow=Wrap  dbl_ovrd=off  block_type=mux
  vout : Outport
  dout : Outport  Port=2
  we_o : Outport  Port=3
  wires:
  Register3/1 -> Concat1/4
  Register2/1 -> Concat1/2
  Constant/1 -> Concat1/3, Concat1/1, Concat/3, Concat/1
  Register1/1 -> Concat/4
  Register/1 -> Concat/2
  [vin] -> vout_choice/2
  Register5/1 -> vout_choice/3
  vout_choice/1 -> vout/1
  Logical2/1 -> Register5/2
  [we] -> Logical2/2, Register4/2
  vin/1 -> [vin], Register5/1
  Register4/1 -> Logical2/1
  [init] -> Register4/3, Register4/1
  dram/1 -> vout_choice/1, we_choice/1, data_choice/1
  [din] -> data_choice/2
  Mux1/1 -> data_choice/3
  [we] -> we_choice/2
  Delay1/1 -> we_choice/3
  we_choice/1 -> we_o/1
  dout_count/1 -> Mux1/1
  [init] -> dout_count/1
  Logical1/1 -> Delay1/1, dout_count/2
  Concat1/1 -> Mux1/3
  Concat/1 -> Mux1/2
  Delay/1 -> Logical1/2
  Logical/1 -> Logical1/1, Delay/1
  Relational3/1 -> Logical/1, Register3/2
  Relational2/1 -> Register2/2
  Relational1/1 -> Register1/2
  Relational/1 -> Register/2
  con3/1 -> Relational3/2
  con2/1 -> Relational2/2
  con1/1 -> Relational1/2
  con0/1 -> Relational/2
  input_count/1 -> Relational3/1, Relational2/1, Relational1/1, Relational/1
  din/1 -> [din], Register3/1, Register2/1, Register1/1, Register/1
  we/1 -> [we], Logical/2, input_count/2
  init/1 -> [init], input_count/1
  data_choice/1 -> dout/1

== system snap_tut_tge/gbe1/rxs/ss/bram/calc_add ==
  note: If reading/writing words smaller than 32 bits, change address so that addressing is big endian instead of little, otherwise pass through
  note: Use behavioural HDL so that gets optimised to minimum logic
  in : Inport
  add_sub : xbsIndex_r4/AddSub  mode=Subtraction  use_carryin=off  use_carryout=off  en=off  latency=0  precision=User Defined  arith_type=Unsigned  n_bits=max(1, log2(32/data_width))  bin_pt=0  quantization=Truncate  overflow=Wrap  use_behavioral_HDL=on  hw_selection=Fabric  pipelined=off  dbl_ovrd=off  block_type=addsub
  concat : xbsIndex_r4/Concat  num_inputs=2  dbl_ovrd=off  block_type=concat
  const : xbsIndex_r4/Constant  const=max(0, 32/data_width-1)  gui_display_data_type=Fixed-point  arith_type=Unsigned  n_bits=max(1, log2(32/data_width))  bin_pt=0  preci_type=Single  exp_width=8  frac_width=24  explicit_period=on  period=sample_rate  equ=P=C  opselect=C  inp2=PCIN>>17  opr=+  inp1=P  carry=CIN  dbl_ovrd=off  block_type=constant
  convert_addr : xbsIndex_r4/Convert  gui_display_data_type=Fixed-point  arith_type=Unsigned  n_bits=addr_width  bin_pt=0  float_type=Single  exp_bits=8  fraction_bits=24  quantization=Truncate  overflow=Wrap  en=off  latency=0  pipeline=off  dbl_ovrd=off  block_type=convert
  lsw : xbsIndex_r4/Slice  nbits=max(1, log2(32/data_width))  boolean_output=off  mode=Lower Bit Location + Width  bit1=0  base1=MSB of Input  bit0=0  base0=LSB of Input  dbl_ovrd=off  block_type=slice
  manipulate : xbsIndex_r4/Constant  const=min(1, floor(32/data_width) - 1)  gui_display_data_type=Fixed-point  arith_type=Unsigned  n_bits=1  bin_pt=0  preci_type=Single  exp_width=8  frac_width=24  explicit_period=on  period=sample_rate  equ=P=C  opselect=C  inp2=PCIN>>17  opr=+  inp1=P  carry=CIN  dbl_ovrd=off  block_type=constant
  msw : xbsIndex_r4/Slice  nbits=addr_width - max(1, log2(32/data_width))  boolean_output=off  mode=Upper Bit Location + Width  bit1=0  base1=MSB of Input  bit0=0  base0=LSB of Input  dbl_ovrd=off  block_type=slice
  mux : xbsIndex_r4/Mux  inputs=2  en=off  latency=0  precision=Full  arith_type=Unsigned  n_bits=16  bin_pt=14  quantization=Truncate  overflow=Wrap  dbl_ovrd=off  block_type=mux
  out : Outport
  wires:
  in/1 -> convert_addr/1
  add_sub/1 -> concat/2
  msw/1 -> concat/1
  concat/1 -> mux/3
  manipulate/1 -> mux/1
  mux/1 -> out/1
  lsw/1 -> add_sub/2
  const/1 -> add_sub/1
  convert_addr/1 -> lsw/1, msw/1, mux/2

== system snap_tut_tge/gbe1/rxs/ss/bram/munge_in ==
  din : Inport
  join : Subsystem  AncestorBlock=casper_library_flow_control/bus_create  mask(bus_create){inputNum=4}
      mask prompts: inputNum "Number of inputs:"
      mask init:
      | bus_create_init(gcb,...
      |     'inputNum', inputNum);
  reinterpret : xbsIndex_r4/Reinterpret  force_arith_type=on  arith_type=Unsigned  force_bin_pt=on  bin_pt=0  block_type=reinterpret
  reinterpret_out : xbsIndex_r4/Reinterpret  force_arith_type=on  arith_type=Unsigned  force_bin_pt=on  bin_pt=0  block_type=reinterpret
  split : Subsystem  AncestorBlock=casper_library_flow_control/bus_expand  mask(bus_expand){mode=divisions of arbitrary size, outputNum=1, outputWidth=[32 32 32 32], outputBinaryPt=[0 0 0 0], outputArithmeticType=[0 0 0 0], show_format=off, outputToWorkspace=off, variablePrefix=out, outputToModelAsWell=on}
      mask prompts: outputNum "Number of outputs:"; outputWidth "Output width [msb ... lsb]:"; outputBinaryPt "Output binary point position [msb ... lsb]:"; outputArithmeticType "Output arithmetic type (ufix=0, fix=1, bool=2) [msb ... lsb]:"; show_format "Print format string?"; outputToWorkspace "Output to workspace?"; variablePrefix "Variable name prefix:"; outputToModelAsWell "Output to model as well?"
      mask help: Expands a 'bus' made using a bus_create or Xilinx concat block. The input will be divided into the specified number of outputs with the specified arithmetic types. Divisions are made from most significant bit.
      mask init:
      | bus_expand_init(gcb,...
      |     'mode', mode, ...
      |     'outputNum', outputNum, ...
      |     'outputWidth', outputWidth, ...
      |     'outputBinaryPt', outputBinaryPt, ...
      |     'outputArithmeticType', outputArithmeticType, ...
      |     'show_format', show_format, ...
      |     'outputToWorkspace', outputToWorkspace, ...
      |     'variablePrefix', variablePrefix, ...
      |     'outputToModelAsWell', outputToModelAsWell);
  dout : Outport
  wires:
  reinterpret_out/1 -> dout/1
  din/1 -> reinterpret/1
  reinterpret/1 -> split/1(bus_in)
  join/1(bus_out) -> reinterpret_out/1
  split/4(lsb_out1) -> join/1(in1)
  split/3(out2) -> join/2(in2)
  split/2(out3) -> join/3(in3)
  split/1(msb_out4) -> join/4(in4)

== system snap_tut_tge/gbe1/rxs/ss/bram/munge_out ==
  din : Inport
  join : Subsystem  AncestorBlock=casper_library_flow_control/bus_create  mask(bus_create){inputNum=4}
      mask prompts: inputNum "Number of inputs:"
      mask init:
      | bus_create_init(gcb,...
      |     'inputNum', inputNum);
  reinterpret : xbsIndex_r4/Reinterpret  force_arith_type=on  arith_type=Unsigned  force_bin_pt=on  bin_pt=0  block_type=reinterpret
  reinterpret_out : xbsIndex_r4/Reinterpret  force_arith_type=on  arith_type=Unsigned  force_bin_pt=on  bin_pt=0  block_type=reinterpret
  split : Subsystem  AncestorBlock=casper_library_flow_control/bus_expand  mask(bus_expand){mode=divisions of arbitrary size, outputNum=1, outputWidth=[32 32 32 32], outputBinaryPt=[0 0 0 0], outputArithmeticType=[0 0 0 0], show_format=off, outputToWorkspace=off, variablePrefix=out, outputToModelAsWell=on}
      mask prompts: outputNum "Number of outputs:"; outputWidth "Output width [msb ... lsb]:"; outputBinaryPt "Output binary point position [msb ... lsb]:"; outputArithmeticType "Output arithmetic type (ufix=0, fix=1, bool=2) [msb ... lsb]:"; show_format "Print format string?"; outputToWorkspace "Output to workspace?"; variablePrefix "Variable name prefix:"; outputToModelAsWell "Output to model as well?"
      mask help: Expands a 'bus' made using a bus_create or Xilinx concat block. The input will be divided into the specified number of outputs with the specified arithmetic types. Divisions are made from most significant bit.
      mask init:
      | bus_expand_init(gcb,...
      |     'mode', mode, ...
      |     'outputNum', outputNum, ...
      |     'outputWidth', outputWidth, ...
      |     'outputBinaryPt', outputBinaryPt, ...
      |     'outputArithmeticType', outputArithmeticType, ...
      |     'show_format', show_format, ...
      |     'outputToWorkspace', outputToWorkspace, ...
      |     'variablePrefix', variablePrefix, ...
      |     'outputToModelAsWell', outputToModelAsWell);
  dout : Outport
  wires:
  reinterpret_out/1 -> dout/1
  din/1 -> reinterpret/1
  reinterpret/1 -> split/1(bus_in)
  join/1(bus_out) -> reinterpret_out/1
  split/4(lsb_out1) -> join/1(in1)
  split/3(out2) -> join/2(in2)
  split/2(out3) -> join/3(in3)
  split/1(msb_out4) -> join/4(in4)

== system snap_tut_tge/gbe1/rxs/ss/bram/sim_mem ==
  addr : Inport
  data : Inport  Port=2
  we : Inport  Port=3
  Data Type Conversion : DataTypeConversion  OutDataTypeStr=single
  Data Type Conversion1 : DataTypeConversion  OutDataTypeStr=double
  Data Type Conversion2 : DataTypeConversion  OutDataTypeStr=boolean
  sfunc : M-S-Function  FunctionName=shared_bram_sim_sfunc  Parameters=depth_bits, latency, init_vals  mask{depth_bits=addr_width, latency=csp_latency, init_vals=init_vals}
      mask prompts: depth_bits "Depth (2^?):"; latency "Latency (>=1):"; init_vals "Initial values:"
  sim_addr : xbsIndex_r4/Gateway Out  inherit_from_input=off  hdl_port=off  rows=1  columns=1  UseAsDAC=off  DACChannel='1'  interface=None  automatic_assignment=on  address_offset=hex2dec('00')  intf_name=''  intf_description=''  timing_constraint=None  locs_specified=off  LOCs={}  io_standard={}  block_type=gatewayout
  sim_data : xbsIndex_r4/Gateway Out  inherit_from_input=off  hdl_port=off  rows=1  columns=1  UseAsDAC=off  DACChannel='1'  interface=None  automatic_assignment=on  address_offset=hex2dec('00')  intf_name=''  intf_description=''  timing_constraint=None  locs_specified=off  LOCs={}  io_standard={}  block_type=gatewayout
  sim_we : xbsIndex_r4/Gateway Out  inherit_from_input=off  hdl_port=off  rows=1  columns=1  UseAsDAC=off  DACChannel='1'  interface=None  automatic_assignment=on  address_offset=hex2dec('00')  intf_name=''  intf_description=''  timing_constraint=None  locs_specified=off  LOCs={}  io_standard={}  block_type=gatewayout
  data_out : Outport
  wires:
  addr/1 -> sim_addr/1
  data/1 -> sim_data/1
  we/1 -> sim_we/1
  sim_addr/1 -> Data Type Conversion/1
  sim_data/1 -> Data Type Conversion1/1
  sim_we/1 -> Data Type Conversion2/1
  Data Type Conversion/1 -> sfunc/1  "addr"
  Data Type Conversion1/1 -> sfunc/2  "data_in"
  Data Type Conversion2/1 -> sfunc/3  "we"
  sfunc/1 -> data_out/1  "output"
